[IBIS Ver]   4.1
[File Name]   sprm383.ibs
[File Rev]   0.1
[Date]   Feb 2007
[Source]   From Optimal Corporation's PakSi-E result.
[Notes]   -Alpha Version
   -PORz Buffer model does not exist, therefore the original
   model was substituted with IHHV33TP18.
   - RIOCLK(N|P) buffer model does not exixt, therefore the
   origional model was substuted for ILVDS18G
[Disclaimer]   This information is for modeling purpose only, and
   is not guaranteed. The information is subject to
   change  without notice.
[Copyright]   Texas Instruments
|   Component   c6472
[Component]   c6472
[Manufacturer]  Texas Instruments.
[Package]
|variable   typ   min   max
R_pkg   8.85E-01   1.98E-01   2.21E+00
L_pkg   2.11E-09   9.58E-10   4.24E-09
C_pkg   1.30E-12   6.99E-13   2.18E-12
[Pin]   signal_name   model_name   R_pin   L_pin   C_pin
  A11   BEA02   BSSTL18GFZ   1.02E+00   2.47E-09   1.40E-12
  A12   BEA01   BSSTL18GFZ   1.07E+00   2.61E-09   1.40E-12
  A13   BED16   BSSTL18GFZ   1.09E+00   2.52E-09   1.45E-12
  A15   BED18   BSSTL18GFZ   1.25E+00   2.69E-09   1.53E-12
  A16   BED22   BSSTL18GFZ   1.19E+00   2.66E-09   1.48E-12
  A17   BED26   BSSTL18GFZ   1.35E+00   2.77E-09   1.60E-12
  A24   EMU12   BT3325ETHYPUFZSCP18  1.40E+00   3.06E-09   1.58E-12
  A26   EMU18   BT3325ETHYPUFZSCP18  1.44E+00   3.04E-09   1.62E-12
  A27   EMU0   BT3325ETHYPUFZSCP18  1.47E+00   3.23E-09   1.65E-12
  A3   BSDDQM0   BSSTL18GFZ   1.62E+00   3.42E-09   1.72E-12
  A4   BCS0z   BSSTL18GFZ   1.45E+00   3.17E-09   1.62E-12
  A6   BBA2   BSSTL18GFZ   1.28E+00   2.75E-09   1.53E-12
  A7   BEA11   BSSTL18GFZ   1.26E+00   2.74E-09   1.55E-12
  A8   BEODT0   BSSTL18GFZ   1.25E+00   3.00E-09   1.52E-12
  A9   BEA06   BSSTL18GFZ   1.17E+00   2.48E-09   1.46E-12
  AA1   TR02   BT3350CTHYPDFZP18   1.49E+00   3.13E-09   1.65E-12
  AA2   CLKB2   BT3350CTHYPDFZP18   1.19E+00   2.81E-09   1.48E-12
  AA25   URSOC   BT3350CTHYPDFZP18   2.60E-01   1.12E-09   8.99E-13
  AA26   UXENBz   BT3350CTHYPUFZP18   4.04E-01   1.50E-09   9.91E-13
  AA27   URDATA2   BT3350CTHYPDFZP18   6.21E-01   1.78E-09   1.14E-12
  AA28   URDATA1   BT3350CTHYPDFZP18   7.66E-01   2.03E-09   1.24E-12
  AA29   URDATA0   BT3350CTHYPDFZP18   9.87E-01   2.55E-09   1.35E-12
  AA3   TX10   BT3350CTHYPDFZP18   8.28E-01   1.98E-09   1.27E-12
  AA4   TR25   BT3350CTHYPDFZP18   5.19E-01   1.61E-09   1.07E-12
  AA5   TX21   BT3350CTHYPDFZP18   2.60E-01   1.09E-09   9.19E-13
  AB25   URDATA5   BT3350CTHYPDFZP18   2.84E-01   1.09E-09   9.11E-13
  AB26   URDATA4   BT3350CTHYPDFZP18   4.81E-01   1.37E-09   1.05E-12
  AB27   URDATA3   BT3350CTHYPDFZP18   6.19E-01   1.75E-09   1.13E-12
  AB3   TR11   BT3350CTHYPDFZP18   9.37E-01   2.17E-09   1.32E-12
  AB4   TR27   BT3350CTHYPDFZP18   6.29E-01   1.90E-09   1.14E-12
  AB5   TR20   BT3350CTHYPDFZP18   3.07E-01   1.12E-09   9.40E-13
  AC1   CLKB1   BT3350CTHYPDFZP18   1.76E+00   3.48E-09   1.85E-12
  AC2   TR15   BT3350CTHYPDFZP18   1.55E+00   3.13E-09   1.70E-12
  AC25   URDATA10   BT3350CTHYPDFZP18   2.58E-01   1.17E-09   9.15E-13
  AC26   URDATA9   BT3350CTHYPDFZP18   4.78E-01   1.47E-09   1.04E-12
  AC27   URDATA8   BT3350CTHYPDFZP18   6.24E-01   1.52E-09   1.14E-12
  AC28   URDATA7   BT3350CTHYPDFZP18   8.46E-01   2.10E-09   1.25E-12
  AC29   URDATA6   BT3350CTHYPDFZP18   9.88E-01   2.19E-09   1.33E-12
  AC3   TR10   BT3350CTHYPDFZP18   1.13E+00   2.44E-09   1.45E-12
  AC4   TX24   BT3350CTHYPDFZP18   7.36E-01   1.80E-09   1.21E-12
  AC5   TX23   BT3350CTHYPDFZP18   5.69E-01   1.72E-09   1.08E-12
  AD1   TX16   BT3350CTHYPDFZP18   1.95E+00   3.79E-09   1.96E-12
  AD2   TX15   BT3350CTHYPDFZP18   1.70E+00   3.67E-09   1.80E-12
  AD25   HASz   BT3350CTHYPUFZP18   6.62E-01   1.62E-09   1.18E-12
  AD26   URDATA15   BT3350CTHYPDFZP18   7.33E-01   1.72E-09   1.21E-12
  AD27   URDATA13   BT3350CTHYPDFZP18   8.60E-01   2.21E-09   1.29E-12
  AD28   URDATA12   BT3350CTHYPDFZP18   9.59E-01   2.14E-09   1.36E-12
  AD29   URDATA11   BT3350CTHYPDFZP18   1.04E+00   2.35E-09   1.38E-12
  AD3   TX13   BT3350CTHYPDFZP18   1.24E+00   2.62E-09   1.55E-12
  AD4   TR26   BT3350CTHYPDFZP18   9.22E-01   2.25E-09   1.33E-12
  AD5   TX22   BT3350CTHYPDFZP18   7.43E-01   1.95E-09   1.21E-12
  AE11   MTXD06_RMTXEN1   BT3325ESHYPUFZSCP18   3.59E-01   1.38E-09   9.75E-13
  AE12   MRXDV0_RMCRSDV1   BT3325ESHYPUFZSCP18   3.29E-01   1.32E-09   9.64E-13
  AE15   RGRD10   BHSTLDVG   3.85E-01   1.43E-09   9.88E-13
  AE16   RGTD12   BHSTLDVG   3.61E-01   1.26E-09   9.80E-13
  AE18   RGTD00   BHSTLDVG   5.33E-01   1.52E-09   1.09E-12
  AE19   RGRD03   BHSTLDVG   5.85E-01   1.64E-09   1.12E-12
  AE22   HD08   BT3350CTHYPDFZP18   6.02E-01   1.78E-09   1.16E-12
  AE23   HDS2z   BT3350CTHYPUFZP18   6.71E-01   1.86E-09   1.16E-12
  AE24   HD02   BT3350CTHYPDFZP18   7.50E-01   1.75E-09   1.20E-12
  AE25   HDS1z   BT3350CTHYPUFZP18   8.21E-01   1.85E-09   1.24E-12
  AE26   HRDYz   BT3350CTHYPUFZP18   9.52E-01   2.29E-09   1.33E-12
  AE27   URENBz   BT3350CTHYPUFZP18   9.76E-01   2.16E-09   1.37E-12
  AE3   TX26   BT3350CTHYPDFZP18   1.37E+00   2.84E-09   1.62E-12
  AE4   TR24   BT3350CTHYPDFZP18   1.04E+00   2.10E-09   1.40E-12
  AE5   TR23   BT3350CTHYPDFZP18   8.26E-01   2.11E-09   1.26E-12
  AE6   MACSEL00   BT3350DTHYPDFZSCP18   5.56E-01   1.72E-09   1.10E-12
  AE7   MTXD4RMTXD10STXCLK1 BT3325ESHYPUFZSCP18   3.86E-01   1.23E-09   9.90E-13
  AE8   MCOL0   BT3350CSHYPDFZP18   3.33E-01   1.27E-09   9.73E-13
  AF1   FSA1   BT3350CTHYPDFZP18 2.21E+00 4.21E-09 2.18E-12
  AF10   MCRS0_RMCRSDV0   BT3350CSHYPDFZP18   5.54E-01   1.76E-09   1.08E-12
  AF11   MTXEN0_RMTXEN0   BT3325ESHYPUFZSCP18   4.92E-01   1.65E-09   1.06E-12
  AF12   MRXER0RMRXER0SRXCLK0 BT3325ESHYPUFZSCP18 5.62E-01 1.66E-09 1.11E-12
  AF15   RGRD11   BHSTLDVG   5.79E-01   1.68E-09   1.09E-12
  AF16   RGTD13   BHSTLDVG   5.99E-01   1.64E-09   1.11E-12
  AF17   RGTD02   BHSTLDVG   5.03E-01   1.52E-09   1.13E-12
  AF18   RGMDCLK   BHSTLDVG   7.38E-01   1.96E-09   1.22E-12
  AF19   RGTXCTL0   BHSTLDVG   7.35E-01   1.95E-09   1.20E-12
  AF2   TX11   BT3350CTHYPDFZP18   1.92E+00   3.72E-09   2.01E-12
  AF20   RGRD02   BHSTLDVG   8.19E-01   2.03E-09   1.26E-12
  AF21   RGRD00   BHSTLDVG   8.91E-01   2.22E-09   1.30E-12
  AF22   HD15   BT3350CTHYPDFZP18   9.04E-01   2.34E-09   1.31E-12
  AF23   HD09   BT3350CTHYPDFZP18   8.83E-01   2.08E-09   1.30E-12
  AF24   HCNTL1   BT3350CTHYPDFZP18   9.67E-01   2.39E-09   1.35E-12
  AF25   HD03   BT3350CTHYPDFZP18   1.04E+00   2.41E-09   1.39E-12
  AF26   HCNTL0   BT3350CTHYPDFZP18   1.12E+00   2.73E-09   1.46E-12
  AF27   HRWz   BT3350CTHYPUFZP18   1.17E+00   2.71E-09   1.50E-12
  AF28   HCSz   BT3350CTHYPUFZP18   1.27E+00   2.98E-09   1.56E-12
  AF29   URDATA14   BT3350CTHYPDFZP18   1.33E+00   2.86E-09   1.58E-12
  AF3   TR22   BT3350CTHYPDFZP18   1.47E+00   2.76E-09   1.71E-12
  AF4   TX20   BT3350CTHYPDFZP18   1.22E+00   2.68E-09   1.53E-12
  AF5   MACSEL10   BT3350DTHYPDFZSCP18   8.99E-01   1.95E-09   1.31E-12
  AF6   MACSEL02   BT3350DTHYPDFZSCP18   6.70E-01   1.76E-09   1.16E-12
  AF8   MTXD00_RMTXD00_STXD0   BT3325ESHYPUFZSCP18   5.68E-01   1.65E-09   1.13E-12
  AF9   MTXD03_STXSYNC1   BT3325ESHYPUFZSCP18   5.15E-01   1.50E-09   1.09E-12
  AG1   TR17   BT3350CTHYPDFZP18   2.18E+00   3.91E-09   2.15E-12
  AG10   MRCLK0_SRXCLK1   BT3325ESHYPUFZSCP18   6.80E-01   1.75E-09   1.16E-12
  AG11   MTXD07_STXCLK0   BT3325ESHYPUFZSCP18   7.10E-01   2.13E-09   1.20E-12
  AG12   MRXD1RMRXD1SRXSYNC0 BT3325ESHYPUFZSCP18 6.98E-01 1.83E-09 1.18E-12
  AG15   RGRXC1   BHSTLDVG   7.15E-01   1.91E-09   1.20E-12
  AG16   RGCLK1   BHSTLDVG   7.32E-01   1.91E-09   1.21E-12
  AG17   RGTD11   BHSTLDVG   7.69E-01   1.94E-09   1.24E-12
  AG18   RGMDIO   BHSTLDVG   8.71E-01   2.08E-09   1.28E-12
  AG19   RGTD01   BHSTLDVG   8.88E-01   2.05E-09   1.31E-12
  AG2   TR16   BT3350CTHYPDFZP18   2.02E+00   3.98E-09   2.08E-12
  AG20   RGCLK0   BHSTLDVG   9.69E-01   2.45E-09   1.36E-12
  AG21   RGRD01   BHSTLDVG   1.05E+00   2.27E-09   1.40E-12
  AG23   HD13   BT3350CTHYPDFZP18   1.12E+00   2.51E-09   1.45E-12
  AG24   HD10   BT3350CTHYPDFZP18   1.16E+00   2.50E-09   1.47E-12
  AG25   HD06   BT3350CTHYPDFZP18   1.20E+00   2.75E-09   1.50E-12
  AG26   HD04   BT3350CTHYPDFZP18   1.28E+00   2.90E-09   1.55E-12
  AG27   HD00   BT3350CTHYPDFZP18   1.35E+00   3.02E-09   1.59E-12
  AG28   HINTz   BT3350CTHYPUFZP18   1.48E+00   3.04E-09   1.68E-12
  AG29   HHWIL   BT3350CTHYPUFZP18   1.50E+00   3.27E-09   1.70E-12
  AG3   TX27   BT3350CTHYPDFZP18   1.66E+00   3.76E-09   1.80E-12
  AG4   PROC1   BT3350CTHYPUFZP18   1.18E+00   2.53E-09   1.49E-12
  AG5   MACSEL01   BT3350DTHYPDFZSCP18   1.01E+00   2.34E-09   1.38E-12
  AG6   GMTCLK0RFCLK1SRFCLK1 BT3325ESHYPUFZSCP18 1.22E+00 2.46E-09 1.46E-12
  AG7   MRXD05_RMRXD11   BT3325ESHYPUFZSCP18   7.50E-01   1.72E-09   1.22E-12
  AG8   MTXD02_STXD1   BT3325ESHYPUFZSCP18   7.78E-01   2.09E-09   1.24E-12
  AG9   GMDCLK   BT3350CSHYPUFZP18   7.30E-01   1.94E-09   1.21E-12
  AH10   GMDIO   BT3350CSHYPUFZP18   8.95E-01   2.32E-09   1.30E-12
  AH11   MRXD00_RMRXD00_SRXD0   BT3325ESHYPUFZSCP18   8.76E-01   2.00E-09   1.31E-12
  AH15   RGRD12   BHSTLDVG   9.33E-01   2.46E-09   1.32E-12
  AH16   RGTXCTL1   BHSTLDVG   9.53E-01   2.22E-09   1.35E-12
  AH17   RGTXC1   BHSTLDVG   9.85E-01   2.41E-09   1.37E-12
  AH18   RGTD10   BHSTLDVG   1.04E+00   2.49E-09   1.41E-12
  AH19   RGTXC0   BHSTLDVG   1.10E+00   2.49E-09   1.45E-12
  AH2   TX14   BT3350CTHYPDFZP18   2.11E+00   4.24E-09   2.17E-12
  AH21   RGRXC0   BHSTLDVG   1.19E+00   2.53E-09   1.49E-12
  AH23   HOUT   BT3350DTHYPUFZSCP18   1.26E+00   2.58E-09   1.51E-12
  AH24   HD12   BT3350CTHYPDFZP18   1.35E+00   3.02E-09   1.59E-12
  AH26   HD07   BT3350CTHYPDFZP18   1.50E+00   2.94E-09   1.67E-12
  AH28   HD01   BT3350CTHYPDFZP18   1.66E+00   3.12E-09   1.80E-12
  AH3   TR21   BT3350CTHYPDFZP18   1.77E+00   3.50E-09   1.90E-12
  AH4   LENDIAN   BT3350DTHYPUFZSCP18   1.35E+00   2.94E-09   1.60E-12
  AH5   MACSEL11   BT3350DTHYPDFZSCP18   1.13E+00   2.30E-09   1.47E-12
  AH7   MTXD1RMTXD1STXSYNC0 BT3325ESHYPUFZSCP18 8.93E-01 2.24E-09 1.30E-12
  AH9   MRXD04_RMRXD10   BT3325ESHYPUFZSCP18   8.70E-01   2.12E-09   1.32E-12
  AJ10   MRXD03_SRXSYNC1   BT3325ESHYPUFZSCP18   1.03E+00   1.96E-09   1.38E-12
  AJ11   MRXD02_SRXD1   BT3325ESHYPUFZSCP18   1.07E+00   2.54E-09   1.40E-12
  AJ13   MRXD06_RMRXER1   BT3325ESHYPUFZSCP18   1.16E+00   2.44E-09   1.44E-12
  AJ15   RGRD13   BHSTLDVG   1.07E+00   2.32E-09   1.39E-12
  AJ16   RGRXCTL1   BHSTLDVG   1.09E+00   2.65E-09   1.42E-12
  AJ19   RGTD03   BHSTLDVG   1.36E+00   2.78E-09   1.59E-12
  AJ21   RGRXCTL0   BHSTLDVG   1.41E+00   2.86E-09   1.60E-12
  AJ24   HD14   BT3350CTHYPDFZP18   1.51E+00   3.13E-09   1.68E-12
  AJ26   HD11   BT3350CTHYPDFZP18   1.64E+00   3.19E-09   1.73E-12
  AJ28   HD05   BT3350CTHYPDFZP18   1.82E+00   3.82E-09   1.88E-12
  AJ3   PROC0   BT3350CTHYPUFZP18   1.52E+00   3.05E-09   1.69E-12
  AJ6   MRXD07   BT3325ESHYPUFZSCP18   1.12E+00   2.49E-09   1.43E-12
  AJ7   MTXD05_RMTXD11   BT3325ESHYPUFZSCP18   1.12E+00   2.46E-09   1.42E-12
  AJ9   MTCLK0RFCLK0SRFCLK0 BT3325ESHYPUFZSCP18 1.09E+00 2.30E-09 1.41E-12
  B11   BEA03   BSSTL18GFZ   8.85E-01   2.02E-09   1.33E-12
  B12   BEA00   BSSTL18GFZ   8.54E-01   1.97E-09   1.31E-12
  B13   BED19   BSSTL18GFZ   9.62E-01   2.49E-09   1.36E-12
  B15   BSDDQM2   BSSTL18GFZ   1.21E+00   2.45E-09   1.50E-12
  B16   BSDDQGATE2   BSSTL18GFZ   1.08E+00   2.47E-09   1.43E-12
  B17   BSDDQS3N   BSSTL18GFZ   1.19E+00   2.67E-09   1.49E-12
  B18   BED28   BSSTL18GFZ   1.27E+00   2.80E-09   1.53E-12
  B19   BED31   BSSTL18GFZ   1.30E+00   2.80E-09   1.56E-12
  B2   BED05   BSSTL18GFZ   1.56E+00   2.99E-09   1.78E-12
  B27   EMU9   BT3325ETHYPUFZSCP18   1.07E+00   2.50E-09   1.41E-12
  B28   TMS   IT33THYPUFZP18   1.29E+00   2.87E-09   1.55E-12
  B29   EMU15   BT3325ETHYPUFZSCP18   1.42E+00   3.12E-09   1.61E-12
  B3   BED02   BSSTL18GFZ   1.38E+00   2.63E-09   1.64E-12
  B4   BED00   BSSTL18GFZ   1.29E+00   2.93E-09   1.51E-12
  B6   BBA1   BSSTL18GFZ   1.19E+00   2.51E-09   1.48E-12
  B7   BEA12   BSSTL18GFZ   1.20E+00   2.71E-09   1.50E-12
  B8   BEA10   BSSTL18GFZ   1.06E+00   2.55E-09   1.43E-12
  B9   BEODT1   BSSTL18GFZ   9.71E-01   2.30E-09   1.40E-12
  C1   BED08   BSSTL18GFZ   1.42E+00   2.93E-09   1.63E-12
  C10   BEA07   BSSTL18GFZ   6.58E-01   1.65E-09   1.21E-12
  C11   BEA04   BSSTL18GFZ   6.29E-01   1.85E-09   1.16E-12
  C12   BED17   BSSTL18GFZ   7.62E-01   1.74E-09   1.26E-12
  C13   BSDDQS2N   BSSTL18GFZ   6.93E-01   1.86E-09   1.17E-12
  C14   BED21   BSSTL18GFZ   8.38E-01   1.85E-09   1.29E-12
  C15   BED24   BSSTL18GFZ   8.32E-01   2.16E-09   1.28E-12
  C16   BSDDQM3   BSSTL18GFZ   8.94E-01   2.04E-09   1.32E-12
  C17   BSDDQS3P   BSSTL18GFZ   1.11E+00   2.50E-09   1.39E-12
  C18   BED30   BSSTL18GFZ   1.09E+00   2.49E-09   1.43E-12
  C2   BSDDQGATE0   BSSTL18GFZ   1.35E+00   2.75E-09   1.64E-12
  C24   EMU4   BT3325ETHYPUFZSCP18   9.98E-01   2.23E-09   1.34E-12
  C25   EMU14   BT3325ETHYPUFZSCP18   1.05E+00   2.36E-09   1.39E-12
  C26   EMU5   BT3325ETHYPUFZSCP18   1.04E+00   2.33E-09   1.38E-12
  C27   TCLK   IQ33TTCKP18PUSR50   1.01E+00   2.52E-09   1.35E-12
  C28   TRSTz   IT33THYPDFZP18   1.21E+00   2.49E-09   1.50E-12
  C29   TDO   BT3350DTHYPUFZSCP18   1.31E+00   3.12E-09   1.56E-12
  C3   BED04   BSSTL18GFZ   1.28E+00   2.62E-09   1.58E-12
  C4   BSDDQS0N   BSSTL18GFZ   1.15E+00   2.45E-09   1.43E-12
  C5   BED01   BSSTL18GFZ   1.13E+00   2.52E-09   1.42E-12
  C6   BSDCKE   BSSTL18GFZ   1.03E+00   2.30E-09   1.38E-12
  C7   BBA0   BSSTL18GFZ   8.97E-01   2.07E-09   1.31E-12
  C8   BECLKOUTP   BSSTL18GFZ   8.11E-01   1.98E-09   1.25E-12
  C9   BEA09   BSSTL18GFZ   7.83E-01   1.88E-09   1.25E-12
  D1   BED13   BSSTL18GFZ   1.37E+00   3.07E-09   1.58E-12
  D10   BEA08   BSSTL18GFZ   5.13E-01   1.41E-09   1.12E-12
  D11   BEA05   BSSTL18GFZ   4.96E-01   1.68E-09   1.09E-12
  D13   BSDDQS2P   BSSTL18GFZ   7.33E-01   1.87E-09   1.21E-12
  D14   BED23   BSSTL18GFZ   6.30E-01   1.72E-09   1.16E-12
  D15   BED25   BSSTL18GFZ   6.17E-01   1.69E-09   1.17E-12
  D16   BED27   BSSTL18GFZ   6.94E-01   1.88E-09   1.17E-12
  D17   BED29   BSSTL18GFZ   8.10E-01   2.11E-09   1.32E-12
  D2   BSDDQGATE1   BSSTL18GFZ   1.25E+00   2.69E-09   1.54E-12
  D22   EMU7   BT3325ETHYPUFZSCP18   7.25E-01   1.80E-09   1.18E-12
  D23   EMU3   BT3325ETHYPUFZSCP18   7.21E-01   1.75E-09   1.19E-12
  D24   EMU13   BT3325ETHYPUFZSCP18   7.70E-01   2.00E-09   1.22E-12
  D25   EMU2   BT3325ETHYPUFZSCP18   7.89E-01   2.10E-09   1.23E-12
  D26   EMU16   BT3325ETHYPUFZSCP18   7.13E-01   2.00E-09   1.19E-12
  D27   TDI   IT33THYPUFZP18   8.99E-01   2.25E-09   1.31E-12
  D28   EMU8   BT3325ETHYPUFZSCP18   1.12E+00   2.39E-09   1.44E-12
  D29   EMU1   BT3325ETHYPUFZSCP18   1.30E+00   2.99E-09   1.55E-12
  D3   BED06   BSSTL18GFZ   1.05E+00   2.33E-09   1.46E-12
  D4   BSDDQS0P   BSSTL18GFZ   1.24E+00   2.67E-09   1.52E-12
  D5   BED03   BSSTL18GFZ   8.89E-01   2.04E-09   1.32E-12
  D6   BSDCASz   BSSTL18GFZ   9.10E-01   2.04E-09   1.32E-12
  D7   BSDRASz   BSSTL18GFZ   6.33E-01   1.86E-09   1.18E-12
  D8   BECLKOUTN   BSSTL18GFZ   8.57E-01   2.07E-09   1.28E-12
  D9   BEA13   BSSTL18GFZ   6.04E-01   1.62E-09   1.15E-12
  E13   BED20   BSSTL18GFZ   3.54E-01   1.26E-09   9.99E-13
  E14   BSDDQGATE3   BSSTL18GFZ   3.57E-01   1.20E-09   1.00E-12
  E2   BED12   BSSTL18GFZ   1.09E+00   2.40E-09   1.41E-12
  E20   DDREN   BT3350DTHYPDFZSCP18   8.75E-01   2.05E-09   1.31E-12
  E22   EMU10   BT3325ETHYPUFZSCP18   5.11E-01   1.52E-09   1.05E-12
  E23   EMU6   BT3325ETHYPUFZSCP18   5.74E-01   1.57E-09   1.10E-12
  E24   EMU17   BT3325ETHYPUFZSCP18   5.80E-01   1.76E-09   1.10E-12
  E25   EMU11   BT3325ETHYPUFZSCP18   4.78E-01   1.54E-09   1.05E-12
  E27   UXDATA2   BT3350CTHYPDFZP18   9.53E-01   2.26E-09   1.35E-12
  E28   UXDATA6   BT3350CTHYPDFZP18   1.10E+00   2.55E-09   1.44E-12
  E29   UXDATA7   BT3350CTHYPDFZP18   1.26E+00   3.05E-09   1.52E-12
  E3   BSDDQS1P   BSSTL18GFZ   1.10E+00   2.39E-09   1.44E-12
  E4   BED09   BSSTL18GFZ   7.83E-01   1.91E-09   1.29E-12
  E5   BED07   BSSTL18GFZ   7.67E-01   1.92E-09   1.30E-12
  E8   BSDWEz   BSSTL18GFZ   4.75E-01   1.32E-09   1.08E-12
  E9   BCS1z   BSSTL18GFZ   3.26E-01   1.17E-09   9.83E-13
  F2   BED15   BSSTL18GFZ   9.15E-01   2.33E-09   1.31E-12
  F26   UXDATA1   BT3350CTHYPDFZP18   6.51E-01   1.94E-09   1.17E-12
  F27   UXDATA5   BT3350CTHYPDFZP18   8.71E-01   2.14E-09   1.28E-12
  F28   UXDATA11   BT3350CTHYPDFZP18   1.09E+00   2.45E-09   1.43E-12
  F29   UXSOC   BT3350CTHYPDFZP18   1.24E+00   2.88E-09   1.50E-12
  F3   BSDDQS1N   BSSTL18GFZ   1.03E+00   2.27E-09   1.34E-12
  F4   BED11   BSSTL18GFZ   6.60E-01   1.77E-09   1.21E-12
  F5   BED10   BSSTL18GFZ   5.97E-01   1.50E-09   1.14E-12
  G1   RESETz   IT33THYP18   1.06E+00   2.23E-09   1.37E-12
  G2   CORESEL2   BT3350CTHYPUFZP18   9.22E-01   2.15E-09   1.30E-12
  G25   UXDATA0   BT3350CTHYPDFZP18   3.68E-01   1.24E-09   9.95E-13
  G26   UXDATA4   BT3350CTHYPDFZP18   5.96E-01   1.63E-09   1.12E-12
  G27   UXDATA10   BT3350CTHYPDFZP18   7.83E-01   2.17E-09   1.25E-12
  G28   UXDATA12   BT3350CTHYPDFZP18   9.70E-01   2.17E-09   1.34E-12
  G3   CORESEL1   BT3350CTHYPUFZP18   7.27E-01   1.82E-09   1.18E-12
  G4   BSDDQM1   BSSTL18GFZ   5.99E-01   1.58E-09   1.13E-12
  G5   BED14   BSSTL18GFZ   3.36E-01   1.24E-09   1.02E-12
|  H1   PORz   IHHV33TP18   1.07E+00   2.34E-09   1.39E-12
  H1   PORz   BSSTL18GFZ   1.07E+00   2.34E-09   1.39E-12
  H2   WDOUTz   BT3350CTHYPUFZP18   8.55E-01   2.14E-09   1.27E-12
  H25   UXDATA3   BT3350CTHYPDFZP18   2.72E-01   1.14E-09   9.37E-13
  H26   UXDATA9   BT3350CTHYPDFZP18   5.56E-01   1.60E-09   1.10E-12
  H27   UXCLAV   BT3350CTHYPDFZP18   7.75E-01   1.89E-09   1.21E-12
  H28   UXDATA13   BT3350CTHYPDFZP18   9.63E-01   2.13E-09   1.35E-12
  H29   UXDATA15   BT3350CTHYPDFZP18   1.15E+00   2.63E-09   1.44E-12
  H3   CORESEL0   BT3350CTHYPUFZP18   6.93E-01   1.94E-09   1.16E-12
  J25   UXDATA8   BT3350CTHYPDFZP18   2.34E-01   1.23E-09   9.24E-13
  J26   UXCLK   BT3350CTHYPDFZP18   4.88E-01   1.32E-09   1.06E-12
  J27   UXDATA14   BT3350CTHYPDFZP18   6.87E-01   1.91E-09   1.18E-12
  J28   URCLAV   BT3350CTHYPDFZP18   8.67E-01   2.25E-09   1.30E-12
  J29   URCLK   BT3350CTHYPDFZP18   1.09E+00   2.58E-09   1.40E-12
  J3   LRESETNMIENz   BT3350CTHYPUFZP18   6.78E-01   1.76E-09   1.17E-12
  J4   LRESETz   BT3350CTHYPUFZP18   4.48E-01   1.50E-09   1.02E-12
  J5   RESETSTATz   BT3350CTHYPUFZP18   3.01E-01   1.14E-09   9.88E-13
  K1   BOOTACTIVE   BT3350CTHYPUFZP18   9.65E-01   2.21E-09   1.34E-12
  K2   NMIz   BT3350CTHYPUFZP18   8.22E-01   2.20E-09   1.27E-12
  K26   SDA   BI2CTFZP18   5.36E-01   1.67E-09   1.11E-12
  K27   SYSCLKOUT   BT3350DTHYPUFZSCP18   7.24E-01   1.83E-09   1.21E-12
  K28   CLKIN1   IT33THYPDFZP18   9.12E-01   2.18E-09   1.31E-12
  K3   GP08_BOOTMODE2   BT3350DTHYPUFZSCP18   6.06E-01   1.63E-09   1.14E-12
  K4   GP09_BOOTMODE3   BT3350DTHYPUFZSCP18   4.65E-01   1.49E-09   1.05E-12
  K5   GP03_TSIP1_EN   BT3350DTHYPDFZSCP18   2.50E-01   1.09E-09   9.25E-13
  L1   GP13_CFGGP3   BT3350DTHYPDFZSCP18   9.30E-01   2.04E-09   1.33E-12
  L2   GP14_CFGGP4   BT3350DTHYPDFZSCP18   7.90E-01   1.98E-09   1.26E-12
  L25   SCL   BI2CTFZP18   2.33E-01   1.10E-09   9.17E-13
  L3   GP15_SYSCLKOUTEN   BT3350DTHYPDFZSCP18   5.71E-01   1.51E-09   1.12E-12
  L4   GP07_BOOTMODE1   BT3350DTHYPUFZSCP18   4.30E-01   1.48E-09   1.02E-12
  L5   GP06_BOOTMODE0   BT3350DTHYPUFZSCP18   2.51E-01   1.17E-09   9.10E-13
  M1   GP00_HPI_EN   BT3350DTHYPDFZSCP18   9.10E-01   2.26E-09   1.32E-12
  M2   GP10_CFGGP0   BT3350DTHYPDFZSCP18   7.90E-01   1.87E-09   1.25E-12
  M3   GP02_TSIP0_EN   BT3350DTHYPDFZSCP18   5.72E-01   1.82E-09   1.11E-12
  M4   GP12_CFGGP2   BT3350DTHYPDFZSCP18   4.30E-01   1.44E-09   1.02E-12
  M5   GP04_TSIP2_EN   BT3350DTHYPDFZSCP18   2.56E-01   1.11E-09   9.29E-13
  N3   GP11_CFGGP1   BT3350DTHYPDFZSCP18   6.32E-01   1.62E-09   1.15E-12
  N4   GP05_EMAC1_EN   BT3350DTHYPDFZSCP18   4.16E-01   1.29E-09   1.02E-12
  N5   GP01_UTOPIA_EN   BT3350DTHYPDFZSCP18   2.47E-01   1.22E-09   9.17E-13
  P1   TX07   BT3350CTHYPDFZP18   9.45E-01   2.17E-09   1.32E-12
  P2   TX04   BT3350CTHYPDFZP18   8.05E-01   2.15E-09   1.25E-12
  P3   TX06   BT3350CTHYPDFZP18   5.75E-01   1.64E-09   1.12E-12
  P4   TX03   BT3350CTHYPDFZP18   4.37E-01   1.41E-09   1.03E-12
  P5   TR04   BT3350CTHYPDFZP18   2.23E-01   1.18E-09   9.01E-13
  R1   TX05   BT3350CTHYPDFZP18   1.04E+00   2.28E-09   1.37E-12
  R2   TR05   BT3350CTHYPDFZP18   8.27E-01   2.09E-09   1.27E-12
  R3   TR06   BT3350CTHYPDFZP18   6.06E-01   1.69E-09   1.14E-12
  R4   CLKB0   BT3350CTHYPDFZP18   4.20E-01   1.33E-09   1.01E-12
  R5   TX01   BT3350CTHYPDFZP18   2.05E-01   1.02E-09   8.91E-13
|  T25   RIOCLKN   ICLKRX18G   3.72E-01   1.25E-09   7.44E-13
  T25   RIOCLKN   ILVDS18G   3.72E-01   1.25E-09   7.44E-13
  T3   TR00   BT3350CTHYPDFZP18   7.03E-01   1.93E-09   1.18E-12
  T4   TX02   BT3350CTHYPDFZP18   4.06E-01   1.42E-09   1.02E-12
  T5   FSB1   BT3350CTHYPDFZP18   2.38E-01   1.02E-09   9.07E-13
  U1   TR07   BT3350CTHYPDFZP18   1.13E+00   2.45E-09   1.41E-12
  U2   TX00   BT3350CTHYPDFZP18   9.37E-01   2.10E-09   1.33E-12
|  U25   RIOCLKP   ICLKRX18G   2.89E-01   1.16E-09   6.99E-13
  U25   RIOCLKP   ILVDS18G   2.89E-01   1.16E-09   6.99E-13
  U26   RIOEN   BT3350DTHYPDFZSCP18   4.34E-01   1.48E-09   1.03E-12
  U3   CLKA0   BT3350CTHYPDFZP18   7.27E-01   1.86E-09   1.21E-12
  U4   TR01   BT3350CTHYPDFZP18   4.07E-01   1.36E-09   1.02E-12
  U5   FSB2   BT3350CTHYPDFZP18   1.98E-01   1.09E-09   8.82E-13
  V1   TR03   BT3350CTHYPDFZP18   1.25E+00   2.66E-09   1.48E-12
  V2   FSA0   BT3350CTHYPDFZP18   9.65E-01   2.35E-09   1.34E-12
  V27   TIMO2   BT3350CTHYPDFZP18   6.02E-01   1.97E-09   1.11E-12
  V28   TIMI0   BT3350CTHYPDFZP18   7.42E-01   2.08E-09   1.19E-12
  V29   TIMI1   BT3350CTHYPDFZP18   9.59E-01   1.98E-09   1.32E-12
  V3   CLKA1   BT3350CTHYPDFZP18   7.24E-01   1.89E-09   1.20E-12
  V4   CLKA2   BT3350CTHYPDFZP18   4.10E-01   1.25E-09   1.02E-12
  W25   UXADDR4   BT3350CTHYPDFZP18   2.05E-01   9.58E-10   8.80E-13
  W26   UXADDR3   BT3350CTHYPDFZP18   4.22E-01   1.47E-09   1.01E-12
  W27   UXADDR2   BT3350CTHYPDFZP18   5.67E-01   1.71E-09   1.10E-12
  W28   UXADDR1   BT3350CTHYPDFZP18   7.86E-01   1.80E-09   1.24E-12
  W29   UXADDR0   BT3350CTHYPDFZP18   9.32E-01   2.40E-09   1.29E-12
  W3   FSA2   BT3350CTHYPDFZP18   7.36E-01   1.92E-09   1.20E-12
  W4   TR14   BT3350CTHYPDFZP18   4.70E-01   1.55E-09   1.04E-12
  W5   TR13   BT3350CTHYPDFZP18   2.03E-01   1.10E-09   8.96E-13
  Y1   FSB0   BT3350CTHYPDFZP18   1.45E+00   2.87E-09   1.62E-12
  Y2   TX17   BT3350CTHYPDFZP18   1.08E+00   2.37E-09   1.40E-12
  Y25   URADDR4   BT3350CTHYPDFZP18   2.07E-01   1.01E-09   8.92E-13
  Y26   URADDR3   BT3350CTHYPDFZP18   4.27E-01   1.53E-09   1.02E-12
  Y27   URADDR2   BT3350CTHYPDFZP18   6.20E-01   1.49E-09   1.14E-12
  Y28   URADDR1   BT3350CTHYPDFZP18   7.63E-01   2.05E-09   1.22E-12
  Y29   URADDR0   BT3350CTHYPDFZP18   9.83E-01   2.27E-09   1.35E-12
  Y3   TR12   BT3350CTHYPDFZP18   7.76E-01   1.87E-09   1.22E-12
  Y4   TX12   BT3350CTHYPDFZP18   5.11E-01   1.62E-09   1.07E-12
  Y5   TX25   BT3350CTHYPDFZP18   2.09E-01   9.86E-10   9.04E-13
[Model Selector] BHSTLDVG
|CELL OPERATING AT TWO VOLTAGES.1.5V/1.8V-DUAL SUPPLY
SR00_1P5  Cell operated at 1.5(nom)
SR00_1P8  Cell operated at 1.8(nom)
|   Component OLVDS18G
[Component]   OLVDS18G
[Manufacturer]   Texas Instruments.
[Package]
| variable   typ   min   max
R_pkg   0.000   0.000   0.000
L_pkg   0.000H   0.000H   0.000H
C_pkg   0.000F   0.000F   0.000F
[Pin]  signal_name   model_name   R_pin   L_pin   C_pin
1   A   OLVDS18G
|   Component IT33THYPDFZP18
[Component]   IT33THYPDFZP18
[Manufacturer]   Texas Instruments
[Package]
|  variable   typ   min   max
R_pkg   0   0   0
L_pkg   0   0   0
C_pkg   0   0   0
[Pin]   signal_name   model_name   R_pin   L_pin   C_pin
1   A   IT33THYPDFZP18
|   Component ILVDS18G
[Component]   ILVDS18G
[Manufacturer]   Texas Instruments
[Package]
|  variable   typ   min   max
R_pkg   0   0   0
L_pkg   0   0   0
C_pkg   0   0   0
[Pin]   signal_name   model_name   R_pin   L_pin   C_pin
1   A   ILVDS18G
|   Component BI2CTFZP18
[Component]   BI2CTFZP18
[Manufacturer]   Texas Instruments
[Package]
|  variable   typ   min   max
R_pkg   0   0   0
L_pkg   0   0   0
C_pkg   0   0   0
[Pin]   signal_name   model_name   R_pin   L_pin   C_pin
1   A   BI2CTFZP18
|   Component BHSTLDVG
[Component]   BHSTLDVG
[Manufacturer]   Texas Instruments
[Package]
|  variable   typ   min   max
R_pkg   0   0   0
L_pkg   0   0   0
C_pkg   0   0   0
[Pin]   signal_name   model_name   R_pin   L_pin   C_pin
1   A   BHSTLDVG
|   Component BT3350CSHYPDFZP18
[Component]   BT3350CSHYPDFZP18
[Manufacturer]   Texas Instruments
[Package]
|  variable   typ   min   max
R_pkg   0   0   0
L_pkg   0   0   0
C_pkg   0   0   0
[Pin]   signal_name   model_name   R_pin   L_pin   C_pin
1   A   BT3350CSHYPDFZP18
|   Component IT33THYPUFZP18
[Component]   IT33THYPUFZP18
[Manufacturer]   Texas Instruments
[Package]
|  variable   typ   min   max
R_pkg   0   0   0
L_pkg   0   0   0
C_pkg   0   0   0
[Pin]   signal_name   model_name   R_pin   L_pin   C_pin
1   A   IT33THYPUFZP18
|   Component IQ33TTCKP18PUSR50
[Component]   IQ33TTCKP18PUSR50
[Manufacturer]   Texas Instruments
[Package]
|  variable   typ   min   max
R_pkg   0   0   0
L_pkg   0   0   0
C_pkg   0   0   0
[Pin]   signal_name   model_name   R_pin   L_pin   C_pin
1   A   IQ33TTCKP18PUSR50
|   Component IT33THYP18
[Component]   IT33THYP18
[Manufacturer]   Texas Instruments
[Package]
|  variable   typ   min   max
R_pkg   0   0   0
L_pkg   0   0   0
C_pkg   0   0   0
[Pin]   signal_name   model_name   R_pin   L_pin   C_pin
1   A   IT33THYP18
|   Component BT3350DTHYPUFZSCP18
[Component]   BT3350DTHYPUFZSCP18
[Manufacturer]   Texas Instruments
[Package]
|  variable   typ   min   max
R_pkg   0   0   0
L_pkg   0   0   0
C_pkg   0   0   0
[Pin]   signal_name   model_name   R_pin   L_pin   C_pin
1   A   BT3350DTHYPUFZSCP18
|   Component BT3350DTHYPDFZSCP18
[Component]   BT3350DTHYPDFZSCP18
[Manufacturer]   Texas Instruments
[Package]
|  variable   typ   min   max
R_pkg   0   0   0
L_pkg   0   0   0
C_pkg   0   0   0
[Pin]   signal_name   model_name   R_pin   L_pin   C_pin
1   A   BT3350DTHYPDFZSCP18
|   Component BT3350CTHYPUFZP18
[Component]   BT3350CTHYPUFZP18
[Manufacturer]   Texas Instruments
[Package]
|  variable   typ   min   max
R_pkg   0   0   0
L_pkg   0   0   0
C_pkg   0   0   0
[Pin]   signal_name   model_name   R_pin   L_pin   C_pin
1   A   BT3350CTHYPUFZP18
|   Component BT3350CTHYPDFZP18
[Component]   BT3350CTHYPDFZP18
[Manufacturer]   Texas Instruments
[Package]
|  variable   typ   min   max
R_pkg   0   0   0
L_pkg   0   0   0
C_pkg   0   0   0
[Pin]   signal_name   model_name   R_pin   L_pin   C_pin
1   A   BT3350CTHYPDFZP18
|   Component BT3350CSHYPUFZP18
[Component]   BT3350CSHYPUFZP18
[Manufacturer]   Texas Instruments
[Package]
|  variable   typ   min   max
R_pkg   0   0   0
L_pkg   0   0   0
C_pkg   0   0   0
[Pin]   signal_name   model_name   R_pin   L_pin   C_pin
1   A   BT3350CSHYPUFZP18
|   Component BT3325ETHYPUFZSCP18
[Component]   BT3325ETHYPUFZSCP18
[Manufacturer]   Texas Instruments
[Package]
|  variable   typ   min   max
R_pkg   0   0   0
L_pkg   0   0   0
C_pkg   0   0   0
[Pin]   signal_name   model_name   R_pin   L_pin   C_pin
1   S   BT3325ETHYPUFZSCP18
|   Component BT3325ESHYPUFZSCP18
[Component]   BT3325ESHYPUFZSCP18
[Manufacturer]   Texas Instruments
[Package]
|  variable   typ   min   max
R_pkg   0   0   0
L_pkg   0   0   0
C_pkg   0   0   0
[Pin]   signal_name   model_name   R_pin   L_pin   C_pin
1   A   BT3325ESHYPUFZSCP18
|   Component BSSTL18GFZ
[Component]   BSSTL18GFZ
[Manufacturer]   Texas Instruments
[Package]
|  variable   typ   min   max
R_pkg   0   0   0
L_pkg   0   0   0
C_pkg   0   0   0
[Pin]   signal_name   model_name   R_pin   L_pin   C_pin
1   A   BSSTL18GFZ
| Models and submodels in the file (18): OLVDS18G (Output), IT33THYPDFZP18 (Input), ILVDS18G (Input), BI2CTFZP18 (I/O_open_drain), SR00_1P5 (I/O), SR00_1P8 (I/O), BT3350CSHYPDFZP18 (I/O), IT33THYPUFZP18 (Input), IQ33TTCKP18PUSR50 (Input), IT33THYP18 (Input), BT3350DTHYPUFZSCP18 (I/O), BT3350DTHYPDFZSCP18 (I/O), BT3350CTHYPUFZP18 (I/O), BT3350CTHYPDFZP18 (I/O), BT3350CSHYPUFZP18 (I/O), BT3325ETHYPUFZSCP18 (I/O), BT3325ESHYPUFZSCP18 (I/O), BSSTL18GFZ (I/O)
